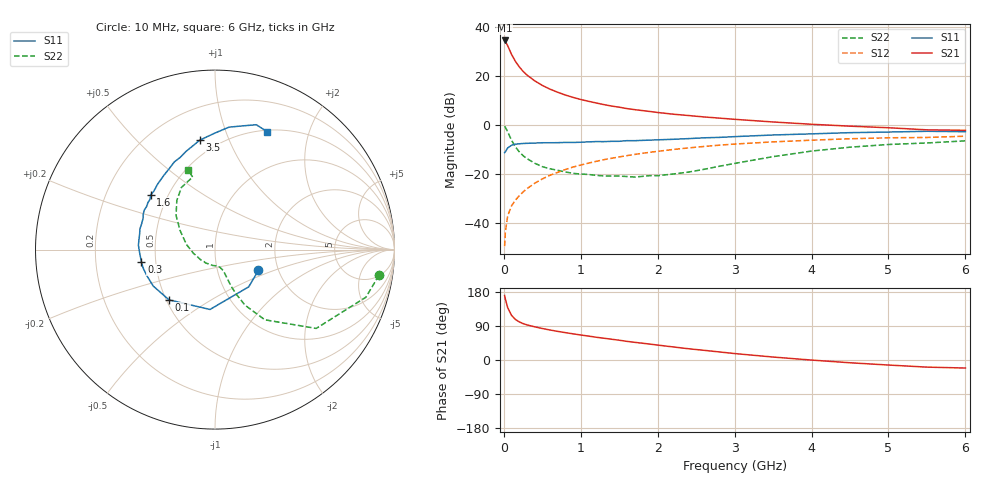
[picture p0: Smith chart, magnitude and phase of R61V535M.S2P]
! SIEMENS Small Signal Semiconductors
! BFR193
! Si NPN RF Bipolar Junction Transistor in SOT23
! VCE = 1.5 V  IC = 35 mA
! Common Emitter S-Parameters:  May  1996
# GHz  S  MA  R  50
!  f  S11  S21  S12  S22
! GHz  MAG  ANG  MAG  ANG  MAG  ANG  MAG  ANG
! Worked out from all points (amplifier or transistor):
!   36 points, 10 MHz to 6 GHz, reference 50 ohm
!   highest |S21| = 34.4 dB at 10 MHz (marker M1)
!   |S21| within 3 dB of that: start of sweep to 62.14 MHz
!   unconditionally stable (mu >= 1): 392.2 MHz to 2.041 GHz
!   at 250 MHz: K = 0.94, MSG = 24.6 dB, |S12| = -27.5 dB
!   at 1.4 GHz: K = 1.03, MAG = 9.7 dB, |S12| = -13.7 dB
!   at 6 GHz: K = 0.96, MSG = 1.2 dB, |S12| = -4.7 dB
!   S11 on the Smith chart (normalised r, x): 10 MHz: 1.58, -0.39; 100 MHz: 0.52, -0.34; 300 MHz: 0.41, -0.07; 1.6 GHz: 0.40, +0.32; 3.5 GHz: 0.40, +0.79; 6 GHz: 0.52, +1.40
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0.01  0.2684 -25.6  52.47 170.0  0.0033 84.6  0.9245 -8.9
0.02  0.2799 -47.9  50.45 160.5  0.0065 77.9  0.8819 -17.5
0.05  0.3347 -94.8  41.01 138.2  0.0137 68.7  0.7148 -37.9
0.1  0.3795 -132.4  27.28 117.8  0.022 65.4  0.4799 -54.6
0.15  0.3997 -149.5  19.64 107.0  0.0287 67.0  0.3525 -61.6
0.2  0.4064 -158.9  15.2 100.7  0.0353 68.9  0.2799 -64.3
0.25  0.4132 -165.4  12.29 96.1  0.0422 70.0  0.2329 -65.9
0.3  0.4159 -170.5  10.36 92.7  0.0492 71.0  0.2032 -66.5
0.4  0.4208 -178.1  7.876 87.6  0.0635 72.3  0.1634 -67.3
0.5  0.4273 176.7  6.337 83.1  0.0779 72.4  0.1388 -67.9
0.6  0.4274 172.0  5.311 79.2  0.0926 71.6  0.1256 -68.7
0.7  0.4287 168.3  4.591 75.5  0.1063 71.2  0.117 -70.4
0.8  0.434 164.6  4.028 72.2  0.1212 70.0  0.1083 -72.7
0.9  0.4333 160.4  3.606 69.0  0.1363 69.0  0.1012 -74.6
1.1  0.4455 154.1  3.003 63.1  0.1639 66.5  0.0961 -82.1
1.3  0.4503 147.8  2.571 57.5  0.1925 63.7  0.0899 -89.9
1.6  0.4716 139.4  2.132 49.2  0.2329 59.3  0.0873 -106.8
2.2  0.5027 124.4  1.637 34.5  0.311 50.1  0.0982 -144.9
3.5  0.6157 97.9  1.135 7.8  0.4451 29.0  0.2225 151.2
4.5  0.6866 83.5  0.932 -7.3  0.5155 14.9  0.347 127.8
5.5  0.7327 71.7  0.784 -18.8  0.5476 1.1  0.4231 107.1
6  0.7186 66.2  0.767 -21.2  0.5816 -2.9  0.467 108.7
